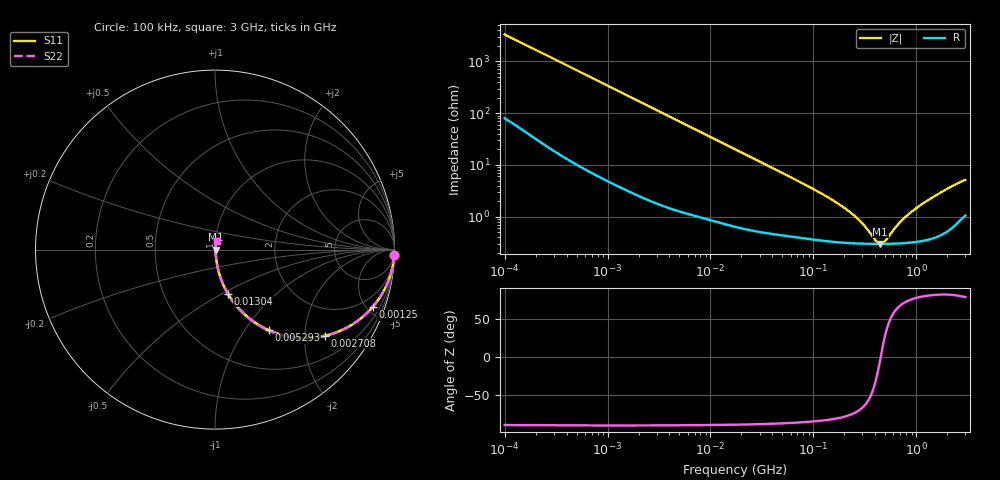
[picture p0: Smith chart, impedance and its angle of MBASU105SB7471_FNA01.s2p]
! MBASU105SB7471_FNA01  S-PARAMETER MODEL  ( Standard Model )
! Model Generated by TAIYO YUDEN Corporation (http://www.ty-top.com)
! Version 1.0
! TAIYO YUDEN Control No. 220601
! Copyright(c) 2017 TAIYO YUDEN CO.,LTD. All Rights Reserved.
! Product Description (link to TY-COMPAS)
! https://ds.yuden.co.jp/TYCOMPAS/or/detail?pn=MBASU105SB7471KFNA01&u=M
! Products Name : Multilayer Ceramic Capacitors
! Characteristics :
!  Capacitance : 470 [pF] , Rated Voltage : 50 [V] , TCC : X7R
!  Case Size : 1.0 x 0.5 / 0.039 x 0.02 [mm/inch] , Thickness : 0.5 / 0.02 [mm/inch]
!  (Conditions: Temperature = 25 [degC] , DC Bias Voltage = 0 [V])
! External Node Assignments :
!  1  o---| |---o  2
! GND o---------o GND
! Frequency Range : 100kHz  -  3GHz  [ 401 STEP ]
# MHZ S RI R 50
! Freq[MHz].  S11 Real  S11 Imag  S21 Real  S21 Imag  S12 Real  S12 Imag  S22 Real  S22 Imag
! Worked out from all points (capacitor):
!   401 points, 100 kHz to 3 GHz, reference 50 ohm
!   read as one part in series: C = 477 pF near 105.3 kHz
!   lowest |Z| = 299 mohm at 445.5 MHz (marker M1)
!   series resonance near 450.9 MHz, so ESL is about 260 pH
!   S11 on the Smith chart (normalised r, x): 100 kHz: 3, -66; 1.25 MHz: 1.08, -5.45; 2.708 MHz: 1.04, -2.53; 5.293 MHz: 1.02, -1.30; 13.04 MHz: 1.01, -0.53; 3 GHz: 1.02, +0.10
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0.1  0.9984 -0.03  0.00163 0.03  0.00163 0.03  0.9984 -0.03
0.259498  0.9928 -0.0764  0.00722 0.0764  0.00722 0.0764  0.9928 -0.0764
0.562235  0.9709 -0.1608  0.0291 0.1608  0.0291 0.1608  0.9709 -0.1608
1.249956  0.8779 -0.3204  0.1221 0.3204  0.1221 0.3204  0.8779 -0.3204
2.708188  0.6138 -0.4792  0.3862 0.4792  0.3862 0.4792  0.6138 -0.4792
3.161081  0.5401 -0.4905  0.4599 0.4905  0.4599 0.4905  0.5401 -0.4905
5.292876  0.3007 -0.4493  0.6993 0.4493  0.6993 0.4493  0.3007 -0.4493
8.202936  0.1564 -0.3521  0.8436 0.3521  0.8436 0.3521  0.1564 -0.3521
13.04487  0.0721 -0.2451  0.9279 0.2451  0.9279 0.2451  0.0721 -0.2451
17.7727  0.0425 -0.1864  0.9575 0.1864  0.9575 0.1864  0.0425 -0.1864
37.52708  0.0132 -0.0914  0.9868 0.0914  0.9868 0.0914  0.0132 -0.0914
97.38194  0.00483 -0.0347  0.9952 0.0347  0.9952 0.0347  0.00483 -0.0347
233.9019  0.00319 -0.0112  0.9968 0.0112  0.9968 0.0112  0.00319 -0.0112
302.6647  0.00304 -0.00654  0.997 0.00654  0.997 0.00654  0.00304 -0.00654
412.3589  0.00297 -0.00143  0.997 0.00143  0.997 0.00143  0.00297 -0.00143
445.5063  0.00297 -0.000193  0.997 0.000193  0.997 0.000193  0.00297 -0.000193
481.3181  0.00298 0.00105  0.997 -0.00105  0.997 -0.00105  0.00298 0.00105
547.5153  0.003 0.00313  0.997 -0.00313  0.997 -0.00313  0.003 0.00313
726.971  0.00312 0.00796  0.9969 -0.00796  0.9969 -0.00796  0.00312 0.00796
1016.304  0.00347 0.0145  0.9965 -0.0145  0.9965 -0.0145  0.00347 0.0145
1886.474  0.00579 0.0318  0.9942 -0.0318  0.9942 -0.0318  0.00579 0.0318
3000  0.0129 0.0492  0.9871 -0.0492  0.9871 -0.0492  0.0129 0.0492
